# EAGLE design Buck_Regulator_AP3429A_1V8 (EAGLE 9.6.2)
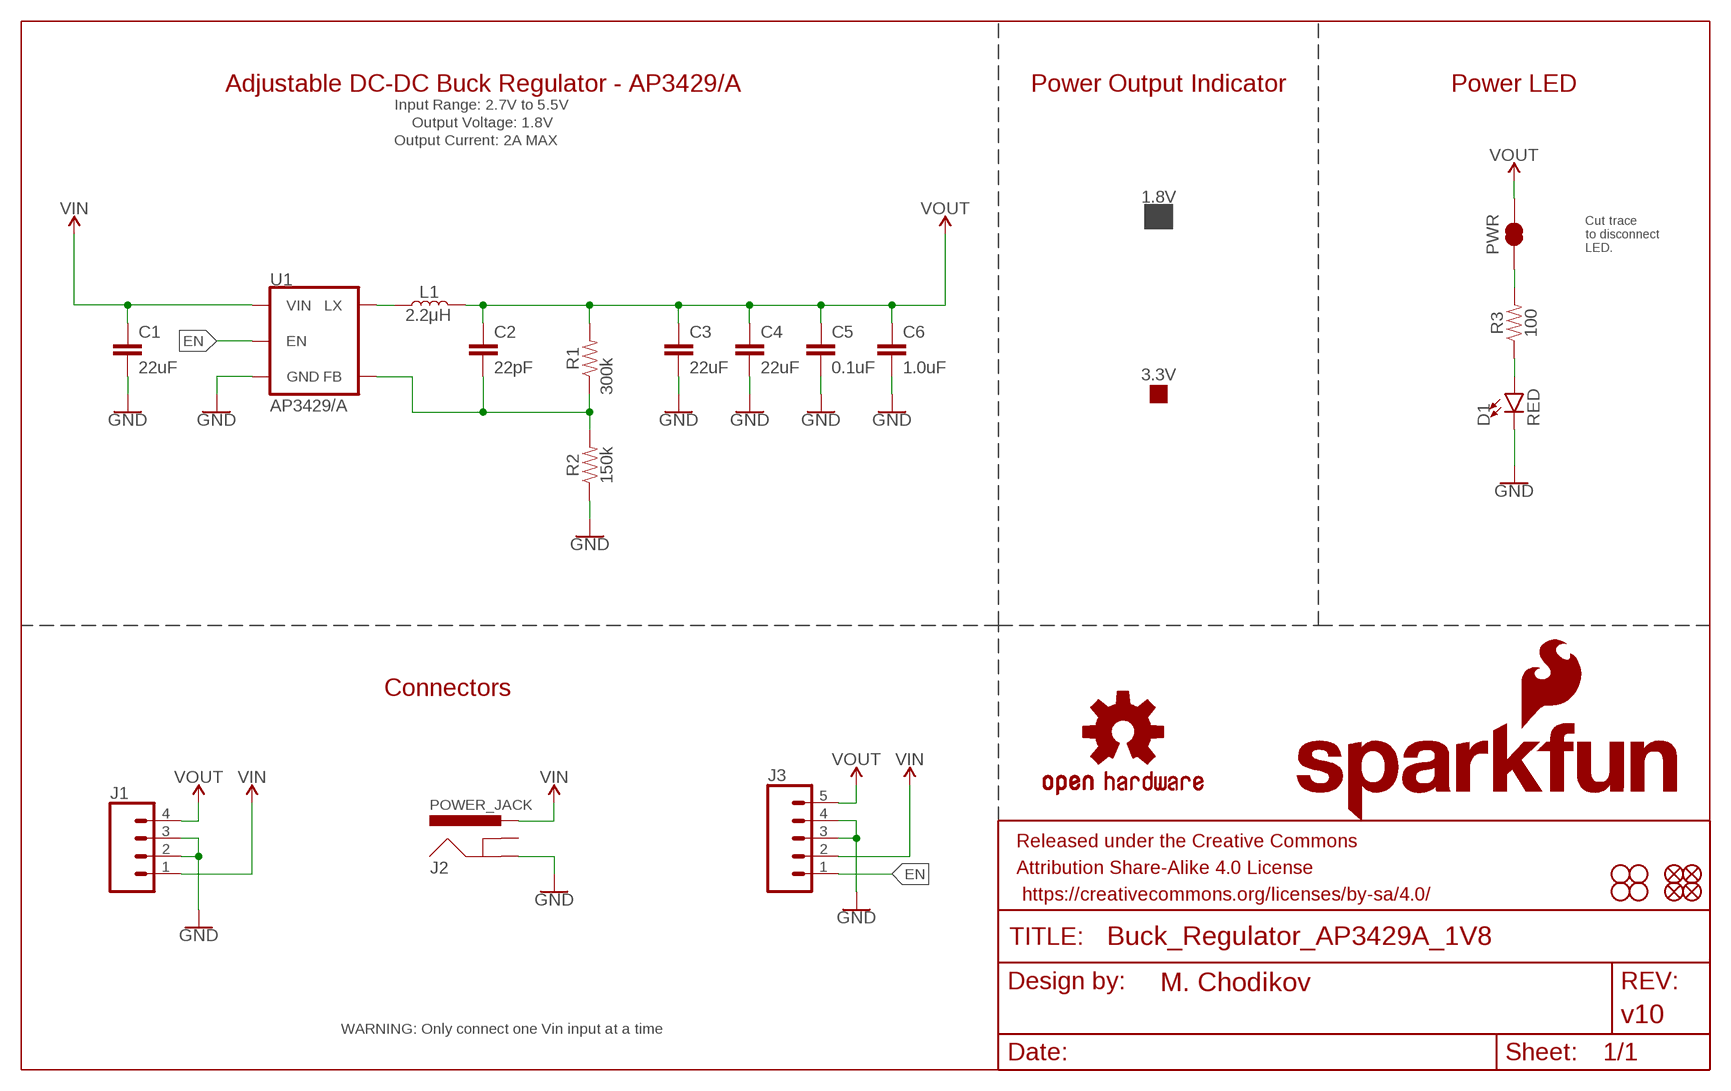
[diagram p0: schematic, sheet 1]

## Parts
1.8V  PROD_ID_PASTE_NO-SILK  [PRODUCT_IDENT_PASTE_NO-SILK]
3.3V  PROD_ID_NO-PASTE_NO_SILK  [PRODUCT_IDENT_NO_NO-SILK]
C1  22uF  22UF-0805-16V-20%  [0805]
C2  22pF  22PF-0402T-16V-10%  [0402-TIGHT]
C3  22uF  22UF-0805-16V-20%  [0805]
C4  22uF  22UF-0805-16V-20%  [0805]
C5  0.1uF  0.1UF-0603-25V-5%  [0603]
C6  1.0uF  1.0UF-0603-16V-10%-X7R  [0603]
D1  RED  LED-RED0603  [LED-0603]
FD1  FIDUCIALUFIDUCIAL  [FIDUCIAL-MICRO]
FD2  FIDUCIALUFIDUCIAL  [FIDUCIAL-MICRO]
FD3  FIDUCIALUFIDUCIAL  [FIDUCIAL-MICRO]
FD4  FIDUCIALUFIDUCIAL  [FIDUCIAL-MICRO]
FRAME1  FRAME-LEDGER  [CREATIVE_COMMONS]
H1  STAND-OFFTIGHT  [STAND-OFF-TIGHT]
H2  STAND-OFFTIGHT  [STAND-OFF-TIGHT]
H3  STAND-OFFTIGHT  [STAND-OFF-TIGHT]
H4  STAND-OFFTIGHT  [STAND-OFF-TIGHT]
J1  Screw Terminal  CONN_04SCREW  [SCREWTERMINAL-3.5MM-4]
J2  POWER_JACKPOWER_JACK_SLOT_COMBO  [POWER_JACK_PTH_SLOT_BOTH]
J3  Breakout Headers  CONN_05NO_SILK  [1X05_NO_SILK]
L1  2.2μH  2.2μH-4X4-2.2μH-3A-45MOHM  [INDUCTOR_4X4MM]
LOGO1  OSHW-LOGOS  [OSHW-LOGO-S]
LOGO2  SFE_LOGO_NAME.1_INCH  [SFE_LOGO_NAME_.1]
LOGO3  SFE_LOGO_FLAME.1_INCH  [SFE_LOGO_FLAME_.1]
PWR  JUMPER-SMT_2_NC_TRACE_SILK  [SMT-JUMPER_2_NC_TRACE_SILK]
R1  300k  300KOHM-0603-1/10W-1%  [0603]
R2  150k  150KOHM-0603-1/10W-1%  [0603]
R3  100  100OHM-0603-1/10W-1%  [0603]
U1  AP3429/A  [SOT23-5]

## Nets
EN: J3.1 U1.1(EN)
GND: C1.2 C3.2 C4.2 C5.2 C6.2 D1.C J1.2 J1.3 J2.GND J3.3 J3.4 R2.1 U1.2(GND)
N$1: L1.P$1 U1.3(LX)
N$2: C2.2 R1.1 R2.2 U1.5(FB)
N$3: PWR.1 R3.2
N$4: D1.A R3.1
VIN: C1.1 J1.1 J2.PWR J3.2 U1.4(VIN)
VOUT: C2.1 C3.1 C4.1 C5.1 C6.1 J1.4 J3.5 L1.P$2 PWR.2 R1.2
Unconnected: J2.GNDBREAK J2.GNDBREAK1(GNDBREAK)

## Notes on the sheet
- Adjustable DC-DC Buck Regulator - AP3429/A | Power Output Indicator | Power LED
- Input Range: 2.7V to 5.5V
- Output Voltage: 1.8V
- Output Current: 2A MAX
- Cut trace
  to disconnect
  LED.
- Connectors
- POWER_JACK
- WARNING: Only connect one Vin input at a time

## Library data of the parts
1.8V = SparkFun-Aesthetics:PROD_ID_PASTE
3.3V = SparkFun-Aesthetics:PROD_ID_NO-PASTE
C1 C3 C4 = SparkFun-Capacitors:22UF: 22µF ceramic capacitors; PROD_ID: CAP-14260
C2 = SparkFun-Capacitors:22PF: 22pF ceramic capacitors; PROD_ID: CAP-14674
C5 = SparkFun-Capacitors:0.1UF: 0.1µF ceramic capacitors; PROD_ID: CAP-08604
C6 = SparkFun-Capacitors:1.0UF: 1µF ceramic capacitors; PROD_ID: CAP-13930
D1 = SparkFun-LED:LED-RED: Red SMD LED; PROD_ID: DIO-00819
FD1-FD4 = SparkFun-Aesthetics:FIDUCIAL: Fiducial Alignment Points
FRAME1 = SparkFun-Aesthetics:FRAME-LEDGER: Schematic Frame - Ledger; DESIGNER: M. Chodikov; REV: v10
H1-H4 = SparkFun-Hardware:STAND-OFF: Stand Off
J1 = SparkFun-Connectors:CONN_04: Multi connection point. Often used as Generic Header-pin footprint for 0.1 inch spaced/style header connections On any of the 0.1 inch spaced packages, you can populate with these: Break Away Headers - Straight (PRT-00116) Break Away Male Headers - Right Angle (PRT-00553) Female Headers (PRT-00115)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; PROD_ID: CONN-14485
J2 = SparkFun-Connectors:POWER_JACK: Power Jack Connector This is the standard 5.5mm barrel jack for power. The PTH is the most common, proven, reliable, footprint. The Slot footprint only works if the mill layer is transmitted to the PCB fab house so be warned. Here are the connectors we sell at SparkFun: DC Barrel Power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
J3 = SparkFun-Connectors:CONN_05: Multi connection point. Often used as Generic Header-pin footprint for 0.1 inch spaced/style header connections On any of the 0.1 inch spaced packages, you can populate with these: Break Away Headers - Straight (PRT-00116) Break Away Male Headers - Right Angle (PRT-00553) Female Headers (PRT-00115)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
L1 = SparkFun-Coils:2.2μH: 2.2μH Inductor; PROD_ID: NDUC-13770
LOGO1 = SparkFun-Aesthetics:OSHW-LOGO: Open-Source Hardware (OSHW) Logo
LOGO2 = SparkFun-Aesthetics:SFE_LOGO_NAME: SparkFun Font Logo
LOGO3 = SparkFun-Aesthetics:SFE_LOGO_FLAME: SparkFun Flame Logo
PWR = SparkFun-Jumpers:JUMPER-SMT_2_NC_TRACE: Normally closed trace jumper
R1 = SparkFun-Resistors:300KOHM: 300kΩ resistor; PROD_ID: RES-10809
R2 = SparkFun-Resistors:150KOHM: 150kΩ resistor; PROD_ID: RES-09117
R3 = SparkFun-Resistors:100OHM: 100Ω resistor; PROD_ID: RES-07863
U1 = SparkFun-IC-Power:AP3429/A: AP3429A DC adjustable buck up to 2A output. Auto cut-off at 2.7V makes this a good option for LiPo and other battery powered circuits.; PROD_ID: IC-14465

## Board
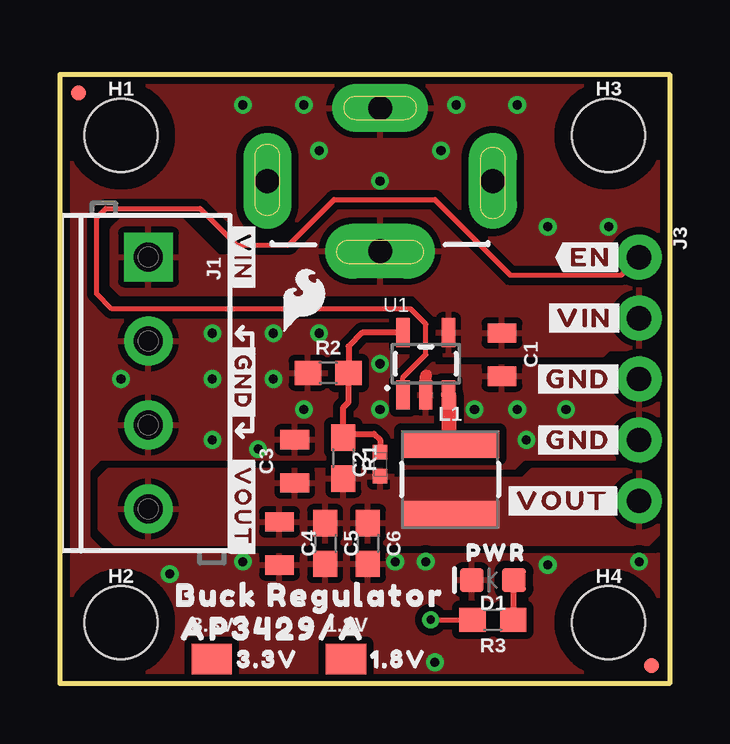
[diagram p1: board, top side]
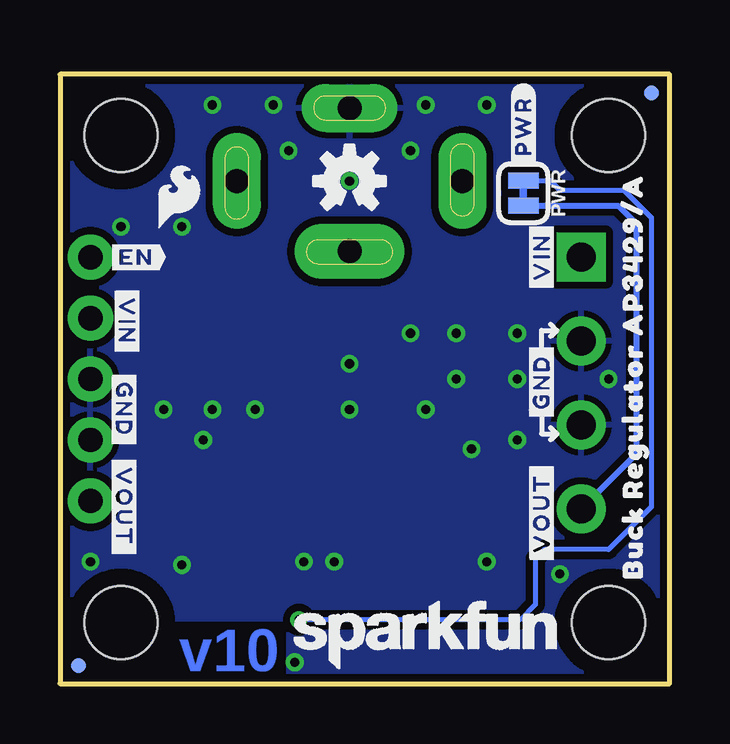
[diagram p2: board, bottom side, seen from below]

Size 25.4 x 25.4 mm. Coordinates in mm from the lower left corner, seen from the top.
Outline: 0,0 0,25.4 25.4,25.4 25.4,0 0,0
Copper layers (1*16): Top 0.035mm / dielectric 1.5mm / Bottom 0.035mm
Design rules "SparkFun-2-Layer-General-JLCPCB": minimum track width 7mil, minimum drill 0.3mm, track to track 7mil, track to pad 7mil, pad to pad 7mil, via to via 7mil, smd to smd 7mil, copper to edge 7mil, drill to drill 7mil, minimum pad ring 7mil, minimum via ring 7mil, stop-mask expansion 3mil, vias tented up to drill 25mil, thermal gap 10mil

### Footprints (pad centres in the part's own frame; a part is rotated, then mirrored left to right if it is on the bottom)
PRODUCT_IDENT_PASTE_NO-SILK = smd 1.676 x 1.27: 1 -0.025,0
PRODUCT_IDENT_NO_NO-SILK = smd 1.676 x 1.27: 1 -0.025,0
0805 = smd 0.8 x 1.2: 1 -0.9,0; 2 0.9,0
0402-TIGHT = smd 0.6 x 0.6: 1 -0.5,0; 2 0.5,0
0603 = smd 1.1 x 1: 1 -0.85,0; 2 0.85,0
LED-0603 = smd 1 x 1: A -0.877,0; C 0.877,0
FIDUCIAL-MICRO = smd 0.635 x 0.635: 1 0,0
STAND-OFF-TIGHT = hole 3.048: 0,0
SCREWTERMINAL-3.5MM-4 = drill 1.2 pad 2.032 square: 1 0,0 | drill 1.2 pad 2.032: 2 3.5,0; 3 7,0; 4 10.5,0
POWER_JACK_PTH_SLOT_BOTH = drill 1 pad 2 long: GND 0,0; GNDBREAK -3.048,4.699; GNDBREAK1 -3.048,-4.699 | drill 1 pad 2.3 long: PWR -5.969,0
1X05_NO_SILK = drill 1.016 pad 1.88: 1 0,0; 2 2.54,0; 3 5.08,0; 4 7.62,0; 5 10.16,0
INDUCTOR_4X4MM = smd 4.089 x 1.143: P$1 0,1.473; P$2 0,-1.473
SMT-JUMPER_2_NC_TRACE_SILK = smd 0.66 x 1.27: 1 -0.521,0; 2 0.521,0
SOT23-5 = smd 0.55 x 1.2: 1 -0.95,-1.3; 2 0,-1.3; 3 0.95,-1.3; 4 0.95,1.3; 5 -0.95,1.3

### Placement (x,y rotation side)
1.8V  11.94,1.02 0 top
3.3V  6.35,1.02 0 top
C1  18.41,13.72 270 top
C2  13.34,9.14 90 top
C3  9.78,9.27 90 top
C4  9.14,5.84 270 top
C5  11.05,5.84 270 top
C6  12.83,5.84 270 top
D1  18.03,4.32 180 top
FD1  24.64,0.76 0 bottom
FD2  24.64,0.76 0 top
FD3  0.76,24.64 0 bottom
FD4  0.76,24.64 0 top
FRAME1  not placed on the board
H1  2.54,22.86 0 top
H2  2.54,2.54 0 top
H3  22.86,22.86 0 top
H4  22.86,2.54 0 top
J1  3.68,17.78 270 top
J2  13.34,24 90 top
J3  24.13,17.78 270 top
L1  16.26,8.51 0 top
LOGO1  13.34,20.95 0 bottom
LOGO2  10.16,2.03 0 bottom
LOGO3  20.45,20.32 0 bottom
PWR  6.1,20.45 270 bottom
R1  11.81,9.4 270 top
R2  11.18,12.95 0 top
R3  18.03,2.67 180 top
U1  15.24,13.34 0 top
U$1  [SFE_LOGO_FLAME_.1]  10.16,16 0 top
U$2  [BUCK_REGULATOR24]  10.41,3.68 0 top
U$3  [AP3429#A25]  8.89,2.29 0 top
U$4  [#VOUT#3431]  20.95,7.62 0 top
U$5  [#GND#3432]  21.59,10.16 0 top
U$6  [#GND#3432]  21.59,12.7 0 top
U$7  [#VIN#3433]  21.84,15.24 0 top
U$8  [#GND#3446]  5.33,12.57 90 bottom
U$9  [#VIN#3445]  22.61,15.11 270 bottom
U$10  [#GND#3446]  22.73,11.43 270 bottom
U$11  [#VOUT#3447]  22.73,7.37 270 bottom
U$12  [#EN#3448]  22.23,17.78 0 bottom
U$13  [#VOUT#3447]  5.33,7.11 90 bottom
U$14  [#PWR#3451]  6.1,23.24 90 bottom
U$15  [#VIN#3445]  5.33,17.78 90 bottom
U$16  [BUCK_REGULATOR_AP3429#A3453]  1.52,12.83 90 bottom
U$17  [ORDERING_INSTRUCTIONS]  not placed on the board
U$19  [1#8V3441]  14.1,1.02 0 top
U$20  [PWR3441]  18.16,5.46 0 top
U$21  [#VOUT#3437]  7.62,7.37 270 top
U$22  [#VIN#3438]  7.62,17.78 270 top
U$23  [3#3V3441]  8.64,1.02 0 top
U$24  [#GND#3439]  7.62,12.57 270 top
U$25  [#EN#3443]  22.1,17.78 0 top

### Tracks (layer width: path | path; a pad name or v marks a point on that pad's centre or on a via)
EN
  Top 0.203: U1.1 14.29,12.77 15.24,13.72 15.24,14.99 14.61,15.62 2.16,15.62 1.52,16.26 1.52,19.43 1.91,19.81 5.84,19.81 7.37,18.29 9.53,18.29 11.42,20.18 15.62,20.18 18.78,17.02 23.37,17.02 J3.1
GND  (via drill 0.38)
  Top 0.203: 15.24,12.83 15.37,12.95
  Top 0.508: U1.2 15.24,12.83
  other vias: 19.43,10.16 24.13,5.08 13.34,20.95 21.08,11.43 20.32,4.95 19.05,11.43 13.34,11.43 13.34,13.34 10.79,14.61 8.89,14.61 8.89,12.7 10.16,11.43 17.27,11.43 8.26,9.78 19.05,24.13 7.62,24.13 6.35,14.61 6.35,10.16 15.24,5.08 7.62,5.08 22.86,19.05 20.32,19.05 6.35,12.7 2.54,12.7 15.62,0.89 15.88,22.23 10.79,22.23 16.51,24.13 10.16,24.13 13.97,5.08 4.57,4.57
  pour Top (isolate 0.305, rank 2): 0,0 0,25.4 25.4,25.4 25.4,0
  pour Bottom (isolate 0.305): 0,0 0,25.4 25.4,25.4 25.4,0
N$1
  Top 0.406: 16.19,10.05 L1.P$1
  Top 0.635: U1.3 16.19,10.05
N$2
  Top 0.178: R1.1 11.86,10.25 | 11.86,10.25
  Top 0.203: 11.86,10.25 12.03,10.41
  Top 0.254: U1.5 12.6,14.63 12.03,14.06 R2.2 12.03,11.73 11.81,11.52 R1.1 | 12.03,10.41 13.08,10.41 13.34,10.16 C2.2
N$3  (via drill 0.35)
  Top 0.203: v15.45,2.67 R3.2
  Bottom 0.203: PWR.1 4.97,20.97 4.57,20.57 1.91,20.57 0.76,19.43 0.76,7.37 2.54,5.59 5.21,5.59 5.59,5.21 5.59,3.3 6.22,2.67 v15.45,2.67
N$4
  Top 0.254: D1.A 18.88,4.29 R3.1
VIN
  pour Top (isolate 0.305): 2.16,18.92 2.16,16.64 2.54,16.26 14.73,16.26 15.75,15.24 15.75,13.97 16,13.72 22.61,13.72 22.86,13.97 24.89,13.97 25.4,14.48 25.4,15.88 24.77,16.51 18.54,16.51 15.24,19.81 11.56,19.81 9.53,17.78 6.6,17.78 4.95,19.43 2.67,19.43
VOUT
  Bottom 0.254: PWR.2 2.15,19.93 1.4,19.18 1.4,9.57 J1.4
  pour Top (isolate 0.305): 1.65,8.51 1.65,6.48 2.29,5.84 13.84,5.84 13.84,8.89 2.03,8.89
  pour Top (isolate 0.305, no thermals): 13.84,5.84 19.3,5.84 19.3,8.51 13.84,8.51
  pour Top (isolate 0.305): 19.3,5.84 24.51,5.84 25.4,6.73 25.4,8.51 25.02,8.89 19.68,8.89 19.3,8.51

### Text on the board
Bottom: v10
Measures: Units in Inches
tDocu: Board thickness is 1.6mm / 2-Layer / 1oz copper | M. Chodikov

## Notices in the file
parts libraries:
SparkFun-Aesthetics: Licensing: Creative Commons ShareAlike 4.0 International - https://creativecommons.org/licenses/by-sa/4.0
SparkFun-Aesthetics: Released under the Creative Commons Attribution Share-Alike 4.0 License
SparkFun-Aesthetics: https://creativecommons.org/licenses/by-sa/4.0
